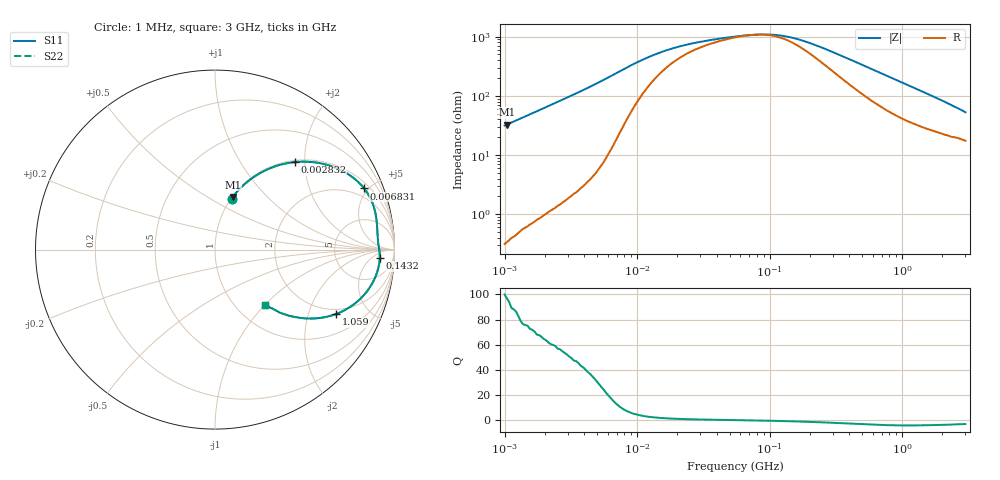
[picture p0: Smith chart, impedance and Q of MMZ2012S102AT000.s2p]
! S-parameter Generated by TDK Corporation
! Copyright(C) 2016 TDK Corporation.
! All Rights Reserved.
! TDK P/N: MMZ2012S102AT000 (Chip Beads)
! Property: |Z|=1000¶ at 100MHz
! Size(LxWxT): 2x1.25x0.85mm, 0.079x0.049x0.033inches
! Model Type: s2p (Touchstone File Format Version 1.0)
! Frequency: DC=Yes Start=1MHz Stop=3000MHz 202points Log-sweep
! Note: This model was converted from impedance.
! Model Generated on May. 16, 2016
! Hash(MD5):
! Port Assignments:
!  1 ---@@@--- 2
! Applicable Conditions:
!  Temperature = 25 degC
!  DC Bias Current = 0 A
!  Small Signal Operation
! Terms and conditions regarding TDK Simulation Models
! (1)This simulation model is being provided solely for informational purposes. Please refer to the specifications of the products in terms of detailed characteristics of such products.
! (2)In no event shall TDK Corporation of any of its subsidiaries be liable for any loss or damage arising, directly or indirectly,
!  From any information contained in this simulation model, including, but not limited to loss or damages arising from any inaccuracies, omissions or errors in connection with such information.
! (3)Any and all copyrights on this simulation model are owned by TDK Corporation.
!  Duplication or redistribution of this simulation model without prior written permission from TDK Corporation is prohibited.
! (4)This simulation model is subject to any modification or change without any prior notice.
! (5)Neither TDK Corporation nor any of its subsidiaries shall make any warranty, express or implied,
!  Including but not limited to the correctness, implied warranties of merchantability and fitness for a particular purpose with respect to this simulation models.
! (6)The use of this simulation model shall be deemed to have consented to the terms and conditions hereof.
# MHz S MA R 50
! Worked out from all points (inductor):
!   201 points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, 1 MHz to 3 GHz, reference 50 ohm
!   read as one part in series: L = 4.99 uH near 1.041 MHz
!   highest Q = 96.9 at 1.041 MHz (marker M1), where L = 5 uH
!   self-resonance near 77.57 MHz
!   S11 on the Smith chart (normalised r, x): 1 MHz: 1.01, +0.63; 2.832 MHz: 1.03, +1.78; 6.831 MHz: 1.34, +4.71; 143.2 MHz: 17, -10; 1.059 GHz: 1.77, -3.06; 3 GHz: 1.35, -1.00
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1  0.2988 72.0  0.9513 -17.4  0.9513 -17.4  0.2988 72.0
1.040844  0.3099 71.4  0.9476 -18.1  0.9476 -18.1  0.3099 71.4
1.682724  0.4638 61.6  0.8794 -27.6  0.8794 -27.6  0.4638 61.6
2.83156  0.6595 47.7  0.7395 -41.3  0.7395 -41.3  0.6595 47.7
3.900413  0.771 38.2  0.6189 -50.4  0.6189 -50.4  0.771 38.2
5.372736  0.8576 28.9  0.483 -59.0  0.483 -59.0  0.8576 28.9
6.83139  0.8981 22.3  0.3803 -63.6  0.3803 -63.6  0.8981 22.3
9.410094  0.9162 15.2  0.2659 -64.2  0.2659 -64.2  0.9162 15.2
14.61624  0.9134 8.9  0.1721 -55.4  0.1721 -55.4  0.9134 8.9
25.59965  0.9089 4.6  0.1192 -37.9  0.1192 -37.9  0.9089 4.6
54.77226  0.9118 1.3  0.09089 -13.4  0.09089 -13.4  0.9118 1.3
95.93103  0.917 -0.9  0.08432 9.8  0.08432 9.8  0.917 -0.9
143.1579  0.9193 -2.9  0.09413 29.5  0.09413 29.5  0.9193 -2.9
213.6344  0.9175 -5.5  0.1235 45.4  0.1235 45.4  0.9175 -5.5
439.1493  0.893 -12.8  0.2356 56.8  0.2356 56.8  0.893 -12.8
581.181  0.8689 -16.8  0.3026 56.2  0.3026 56.2  0.8689 -16.8
800.5644  0.8232 -22.4  0.3945 52.7  0.3945 52.7  0.8232 -22.4
1059.487  0.7646 -28.0  0.4838 47.8  0.4838 47.8  0.7646 -28.0
1402.151  0.6871 -33.8  0.5748 41.7  0.5748 41.7  0.6871 -33.8
1782.824  0.6085 -38.7  0.6484 35.9  0.6484 35.9  0.6085 -38.7
2266.846  0.5218 -43.3  0.7164 30.0  0.7164 30.0  0.5218 -43.3
3000  0.4134 -47.7  0.7841 23.0  0.7841 23.0  0.4134 -47.7
